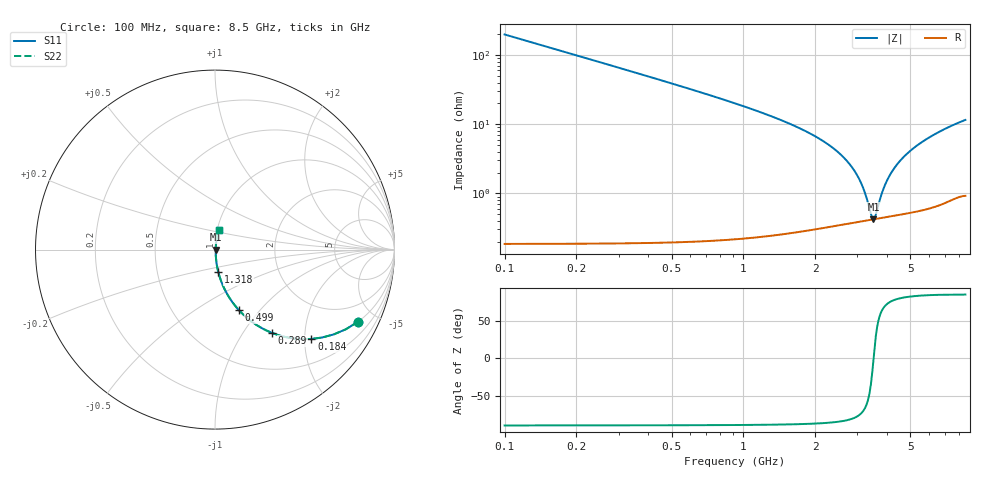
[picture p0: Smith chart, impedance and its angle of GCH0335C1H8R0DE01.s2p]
!Murata Part Number: GCH0335C1H8R0DE01
!These Parameters are Measured in Series Mode Connection
!Data Generated on Mar 13, 2026
!  o--ll--o
!Port1  Port2
!  o------o
!Operation Temp=25[degC], DC Bias Voltage=0[V]
!Freq. Start=100[MHz] Stop=9[GHz] 401[Steps]
# Hz S RI R 50
!Freq.(Hz) S11(Real) S11(Imag) S21(Real) S21(Imag) S12(Real) S12(Imag) S22(Real) S22(Imag)
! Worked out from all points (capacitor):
!   401 points, 100 MHz to 8.5 GHz, reference 50 ohm
!   read as one part in series: C = 8 pF near 142 MHz
!   lowest |Z| = 421 mohm at 3.502 GHz (marker M1)
!   series resonance near 3.507 GHz, so ESL is about 260 pH
!   S11 on the Smith chart (normalised r, x): 100 MHz: 1.00, -3.98; 184 MHz: 1.00, -2.16; 289 MHz: 1.00, -1.37; 499 MHz: 1.00, -0.78; 1.318 GHz: 1.00, -0.26; 8.5 GHz: 1.02, +0.23
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1e8  0.7978 -0.4012  0.2022 0.4012  0.2022 0.4012  0.7978 -0.4012
1.84e8  0.5375 -0.4977  0.4625 0.4977  0.4625 0.4977  0.5375 -0.4977
2.89e8  0.3189 -0.4647  0.6811 0.4647  0.6811 0.4647  0.3189 -0.4647
3.73e8  0.2183 -0.4113  0.7817 0.4113  0.7817 0.4113  0.2183 -0.4113
4.99e8  0.1335 -0.3376  0.8665 0.3376  0.8665 0.3376  0.1335 -0.3376
8.35e8  0.0497 -0.2128  0.9503 0.2128  0.9503 0.2128  0.0497 -0.2128
1.318e9  0.0187 -0.1264  0.9813 0.1264  0.9813 0.1264  0.0187 -0.1264
1.507e9  0.0139 -0.1054  0.9861 0.1054  0.9861 0.1054  0.0139 -0.1054
2.41e9  0.0052 -0.0429  0.9948 0.0429  0.9948 0.0429  0.0052 -0.0429
2.914e9  0.00419 -0.0208  0.9958 0.0208  0.9958 0.0208  0.00419 -0.0208
3.166e9  0.00408 -0.0114  0.9959 0.0114  0.9959 0.0114  0.00408 -0.0114
3.439e9  0.00415 -0.00218  0.9958 0.00218  0.9958 0.00218  0.00415 -0.00218
3.502e9  0.00419 -0.000154  0.9958 0.000154  0.9958 0.000154  0.00419 -0.000154
3.565e9  0.00424 0.00183  0.9958 -0.00183  0.9958 -0.00183  0.00424 0.00183
3.754e9  0.00443 0.0076  0.9956 -0.0076  0.9956 -0.0076  0.00443 0.0076
3.901e9  0.00461 0.0119  0.9954 -0.0119  0.9954 -0.0119  0.00461 0.0119
4.09e9  0.00489 0.0172  0.9951 -0.0172  0.9951 -0.0172  0.00489 0.0172
4.3e9  0.00526 0.0229  0.9947 -0.0229  0.9947 -0.0229  0.00526 0.0229
4.888e9  0.00655 0.0378  0.9934 -0.0378  0.9934 -0.0378  0.00655 0.0378
5.707e9  0.00897 0.0567  0.991 -0.0567  0.991 -0.0567  0.00897 0.0567
7.114e9  0.0149 0.0862  0.9851 -0.0862  0.9851 -0.0862  0.0149 0.0862
8.5e9  0.0219 0.1116  0.9781 -0.1116  0.9781 -0.1116  0.0219 0.1116
